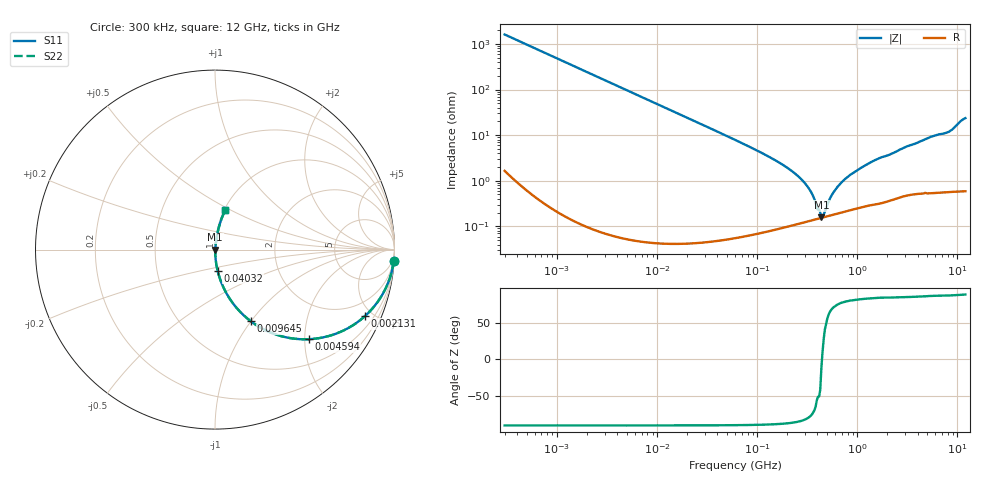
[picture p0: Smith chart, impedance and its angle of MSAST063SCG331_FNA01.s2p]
! MSAST063SCG331_FNA01  S-PARAMETER MODEL  ( General Type )
! Model Generated by TAIYO YUDEN Corporation (http://www.ty-top.com)
! Version 1.0
! TAIYO YUDEN Control No. 160830
! Copyright(c) 2016 TAIYO YUDEN CO.,LTD. All Rights Reserved.
! Product Description (link to TY-COMPAS)
! https://ds.yuden.co.jp/TYCOMPAS/or/detail?pn=MSAST063SCG331JFNA01&u=M
! Products Name : Multilayer Ceramic Capacitors
! Characteristics :
!  Capacitance : 330 pF , Rated Voltage : 25V , TCC : CG / C0G
!  Case Size : 0.6 x 0.3 / 0.024 x 0.012 [mm/inch] , Thickness : 0.3 / 0.012 [mm/inch]
!  (Conditions: Temperature = 25 degC , DC Bias Current/Voltage = 0A / 0V)
! External Node Assignments :
!  1  o---| |---o  2
! GND o---------o GND
! Frequency Range : 0.3MHz  -  12000MHz  [ 401 STEP ]
# MHz S RI R 50
! Freq[MHz].  S11 Real  S11 Imag  S21 Real  S21 Imag  S12 Real  S12 Imag  S22 Real  S22 Imag
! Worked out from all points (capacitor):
!   401 points, 300 kHz to 12 GHz, reference 50 ohm
!   read as one part in series: C = 330 pF near 316.3 kHz
!   lowest |Z| = 157 mohm at 437.6 MHz (marker M1)
!   series resonance near 443.6 MHz, so ESL is about 390 pH
!   S11 on the Smith chart (normalised r, x): 300 kHz: 1, -32; 2.131 MHz: 1.00, -4.53; 4.594 MHz: 1.00, -2.10; 9.645 MHz: 1.00, -1.00; 40.32 MHz: 1.00, -0.24; 12 GHz: 1.01, +0.47
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0.3  0.9961 -0.062  0.00392 0.062  0.00392 0.062  0.9961 -0.062
0.758231  0.9758 -0.1534  0.0242 0.1534  0.0242 0.1534  0.9758 -0.1534
1.769972  0.8812 -0.3234  0.1188 0.3234  0.1188 0.3234  0.8812 -0.3234
2.130602  0.8366 -0.3695  0.1634 0.3695  0.1634 0.3695  0.8366 -0.3695
4.593584  0.5243 -0.4992  0.4757 0.4992  0.4757 0.4992  0.5243 -0.4992
9.644859  0.2001 -0.3996  0.7999 0.3996  0.7999 0.3996  0.2001 -0.3996
10.44266  0.1759 -0.3802  0.8241 0.3802  0.8241 0.3802  0.1759 -0.3802
18.70358  0.0625 -0.2412  0.9375 0.2412  0.9375 0.2412  0.0625 -0.2412
40.32496  0.0143 -0.1169  0.9857 0.1169  0.9857 0.1169  0.0143 -0.1169
60  0.00673 -0.0783  0.9933 0.0783  0.9933 0.0783  0.00673 -0.0783
208.3979  0.00133 -0.018  0.9987 0.018  0.9987 0.018  0.00133 -0.018
286.3882  0.0013 -0.00979  0.9987 0.00979  0.9987 0.00979  0.0013 -0.00979
353.9943  0.00138 -0.00491  0.9986 0.00491  0.9986 0.00491  0.00138 -0.00491
414.98  0.00149 -0.0018  0.9985 0.0018  0.9985 0.0018  0.00149 -0.0018
437.5599  0.00154 -0.000302  0.9985 0.000302  0.9985 0.000302  0.00154 -0.000302
461.3684  0.00159 0.000839  0.9984 -0.000839  0.9984 -0.000839  0.00159 0.000839
585.5907  0.00185 0.0055  0.9981 -0.0055  0.9981 -0.0055  0.00185 0.0055
743.2595  0.0022 0.0103  0.9978 -0.0103  0.9978 -0.0103  0.0022 0.0103
1262.535  0.00333 0.023  0.9967 -0.023  0.9967 -0.023  0.00333 0.023
2088.533  0.00496 0.0367  0.995 -0.0367  0.995 -0.0367  0.00496 0.0367
8064.993  0.0188 0.1136  0.9812 -0.1136  0.9812 -0.1136  0.0188 0.1136
12000  0.0577 0.221  0.9423 -0.221  0.9423 -0.221  0.0577 0.221
